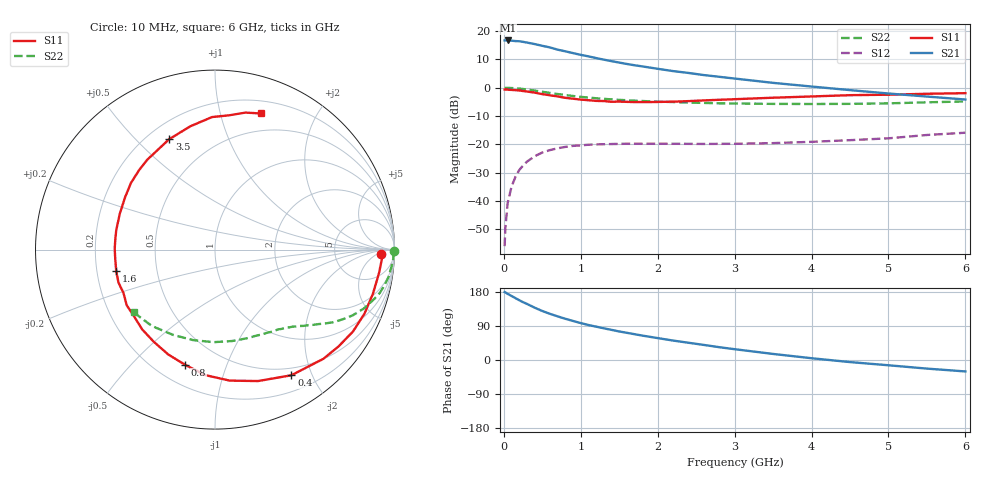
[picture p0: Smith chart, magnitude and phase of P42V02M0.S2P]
! SIEMENS Small Signal Semiconductors
! BFP182
! Si NPN RF Bipolar Junction Transistor in SOT143
! VCE = 2 V  IC = 2 mA
! Common Emitter S-Parameters:  March  1996
# GHz  S  MA  R  50
!  f  S11  S21  S12  S22
! GHz  MAG  ANG  MAG  ANG  MAG  ANG  MAG  ANG
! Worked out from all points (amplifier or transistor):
!   36 points, 10 MHz to 6 GHz, reference 50 ohm
!   highest |S21| = 16.7 dB at 50 MHz (marker M1)
!   |S21| within 3 dB of that: start of sweep to 667.9 MHz
!   unconditionally stable (mu >= 1): 2.159 GHz to 5.977 GHz
!   at 250 MHz: K = 0.13, MSG = 21.8 dB, |S12| = -27.5 dB
!   at 1.4 GHz: K = 0.68, MSG = 14.6 dB, |S12| = -19.9 dB
!   at 6 GHz: K = 1.00, MSG = 5.9 dB, |S12| = -15.9 dB
!   lowest NFmin = 1.10 dB at 450 MHz
!   S11 on the Smith chart (normalised r, x): 10 MHz: 23, -8; 400 MHz: 0.40, -1.71; 800 MHz: 0.32, -0.72; 1.6 GHz: 0.28, -0.10; 3.5 GHz: 0.28, +0.63; 6 GHz: 0.32, +1.35
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0.01  0.9266 -1.6  6.818 179.2  0.0016 88.4  0.9964 -0.6
0.02  0.9315 -3.1  6.818 178.4  0.0034 86.6  0.9944 -1.3
0.05  0.9234 -8.0  6.82 174.5  0.0093 87.6  0.9944 -3.0
0.1  0.9138 -15.6  6.761 169.0  0.0179 80.0  0.9862 -6.1
0.2  0.8941 -30.7  6.606 157.8  0.0353 72.1  0.9655 -11.9
0.25  0.8745 -38.1  6.441 152.6  0.0423 67.7  0.9488 -14.8
0.4  0.8193 -58.7  5.89 138.1  0.0618 57.0  0.8908 -21.7
0.5  0.7706 -71.9  5.485 129.3  0.0719 50.3  0.8493 -25.6
0.6  0.7345 -83.6  5.134 121.8  0.0793 44.5  0.8085 -28.8
0.7  0.7017 -94.3  4.69 115.1  0.0854 40.2  0.7737 -31.5
0.8  0.6631 -104.5  4.385 108.7  0.0903 36.0  0.7425 -33.6
1  0.6168 -123.5  3.797 97.4  0.0961 29.2  0.6901 -37.4
1.1  0.6018 -132.4  3.574 92.3  0.0986 26.9  0.669 -39.0
1.3  0.5815 -147.8  3.127 83.6  0.1008 22.2  0.636 -42.0
1.6  0.5629 -168.0  2.623 71.7  0.1027 17.6  0.6013 -46.0
1.8  0.5587 179.6  2.377 64.4  0.1027 15.8  0.5826 -48.7
2.2  0.567 159.2  1.965 51.3  0.1024 13.1  0.5587 -54.7
2.8  0.6121 133.8  1.558 33.8  0.1022 12.5  0.5306 -65.0
3.5  0.6662 112.5  1.218 16.0  0.1053 13.7  0.5183 -79.3
4.5  0.7386 91.3  0.907 -5.5  0.1187 16.4  0.5188 -103.6
5.5  0.7818 77.5  0.698 -22.7  0.1465 16.8  0.5522 -129.6
6  0.8011 71.2  0.619 -30.2  0.1606 13.8  0.5725 -142.4
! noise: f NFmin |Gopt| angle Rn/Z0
0.45  1.1  0.42  29  0.36
0.9  1.2  0.4  58  0.3
1.8  1.85  0.32  126  0.22
